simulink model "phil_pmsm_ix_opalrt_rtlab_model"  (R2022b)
settings: Solver=ode3  StartTime=0.0  StopTime=inf  FixedStep=Ts  RelTol=1e-3
PostLoadFcn:
  | phil_pmsm_ix_opalrt_rtlab_param;
InitFcn:
  | phil_pmsm_ix_opalrt_rtlab_param;
undefined symbols (not defined in the file or in its folder): af15, arm1_g1, Boost2lvl_SFun, boost_I, boost_V, C, c62c8459, DB, EFPGASIMConfig, eHSBuildReport, eHSx64_Gen4_Machines_IOConfig1, EX, fault_sw, LABv2024, logs, matlab, Min, models, ns, OPAL, phil_pmsm_ix_opalrt_rtlab, phil_pmsm_ix_opalrt_rtlab_ehs, phil_pmsm_ix_opalrt_rtlab_model, phil_pmsm_ix_opalrt_rtlab_param, RT, Step, TE0741_4, Time, Users, v1, vin, vsrc1, vsrc2, vsrc3
libraries: opal_lib x3, rtlab x2, rtio_opalrt_common x1, ehsSchematicEditorSourceLib x1

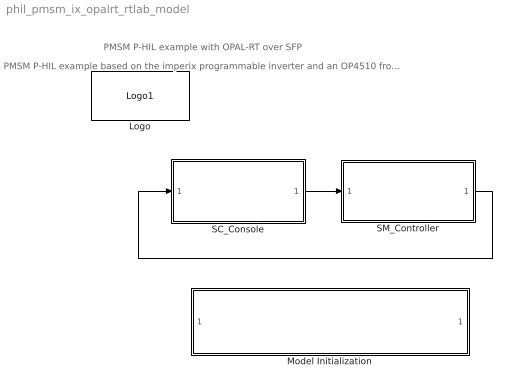
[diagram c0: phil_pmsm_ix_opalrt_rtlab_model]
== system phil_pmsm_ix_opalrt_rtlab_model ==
  note: PMSM P-HIL example based on the imperix programmable inverter and an OP4510 from OPAL-RT.
  note: PMSM P-HIL example with OPAL-RT over SFP
  Logo : opal_lib/Logo1  vide=[]
  Model Initialization : Subsystem  mask(Model Functions){InitFcnX=phil_pmsm_ix_opalrt_rtlab_param;, prel=off, posl=on, inif=on, strf=off}
      mask prompts: InitFcnX "Initialisation"; prel "Preload Function"; posl "PostLoad Function"; inif "InitFcn"; strf "StartFcn"
      mask init:
      | currentBlock = gcb;
      | root = bdroot(currentBlock);
      | 
      | if ~strcmp(get_param(root,'BlockDiagramType'),'library')
      |     if prel==1
      |         set_param(root, 'PreLoadFcn', InitFcnX);
      |     else
      |         set_param(root, 'PreLoadFcn', '');
      |     end
      |     if inif==1
      |         set_param(root, 'InitFcn', InitFcnX);
      |     else
      |         set_param(root, 'InitFcn', '');
      |     end
      |     if strf==1
      |         set_param(root, 'StartFcn', InitFcnX);
      |     else
      |         set_param(root, 'StartFcn', '');
      |     end
      |     if posl==1
      |         set_param(root, 'PostLoadFcn', InitFcnX);
      |     else
      |         set_param(root, 'PostLoadFcn', '');
      |     end
      | end
      | 
      | pos = get_param(currentBlock, 'Position');
      | width = pos(3) - pos(1); height = pos(4) - pos(2);
      | txt = [ upper(root) '\n' '- InitFcn. . . . . '  get_param(root, 'InitFcn') ];
  SC_Console : Subsystem
  SM_Controller : Subsystem
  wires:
  SC_Console/1(to_eHS) -> SM_Controller/1(to_eHS)
  SM_Controller/1(from_eHS) -> SC_Console/1(from_eHS)

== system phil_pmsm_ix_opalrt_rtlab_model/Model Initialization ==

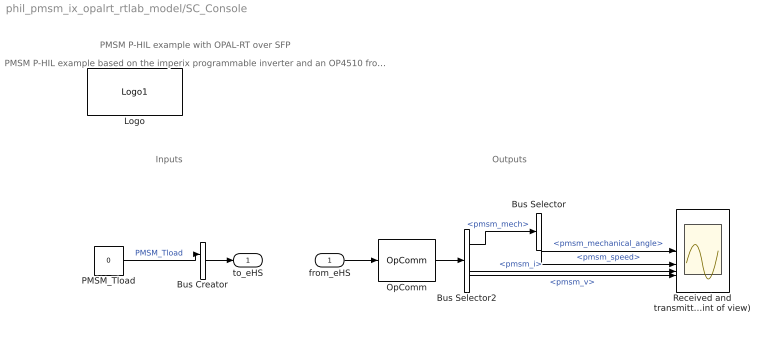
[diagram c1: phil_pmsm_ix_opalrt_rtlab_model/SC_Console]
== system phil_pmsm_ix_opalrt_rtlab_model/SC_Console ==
  note: Inputs
  note: Outputs
  note: PMSM P-HIL example with OPAL-RT over SFP
  note: PMSM P-HIL example based on the imperix programmable inverter and an OP4510 from OPAL-RT.
  from_eHS : Inport  OutDataTypeStr=double
  Bus Creator : BusCreator  Inputs=1
  Bus Selector : BusSelector  OutputSignals=pmsm_mechanical_angle,pmsm_speed
  Bus Selector2 : BusSelector  OutputSignals=pmsm_mech,pmsm_i,pmsm_v
  Logo : opal_lib/Logo1  vide=[]
  OpComm : rtlab/OpComm  nbport=1  groupe_acq=1  subsys_rate=0  st=0  Synchronization=off  Interpolation=off  Threshold=1.0  Missed_Data=off  Sim_Time=off  Samples=off  dynSigOut=off  from_console=0  warning_done=off  writeOpCommFile=off
  PMSM_Tload : Constant  Value=0
  Received and transmitted signals (OP4510 point of view) : Scope  NumInputPorts=4
  to_eHS : Outport  VectorParamsAs1DForOutWhenUnconnected=off
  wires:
  from_eHS/1 -> OpComm/1
  Bus Creator/1 -> to_eHS/1
  OpComm/1 -> Bus Selector2/1
  PMSM_Tload/1 -> Bus Creator/1  "PMSM_Tload"
  Bus Selector2/1 -> Bus Selector/1  "<pmsm_mech>"
  Bus Selector2/2 -> Received and transmitted signals (OP4510 point of view)/3  "<pmsm_i>"
  Bus Selector2/3 -> Received and transmitted signals (OP4510 point of view)/4  "<pmsm_v>"
  Bus Selector/1 -> Received and transmitted signals (OP4510 point of view)/1  "<pmsm_mechanical_angle>"
  Bus Selector/2 -> Received and transmitted signals (OP4510 point of view)/2  "<pmsm_speed>"

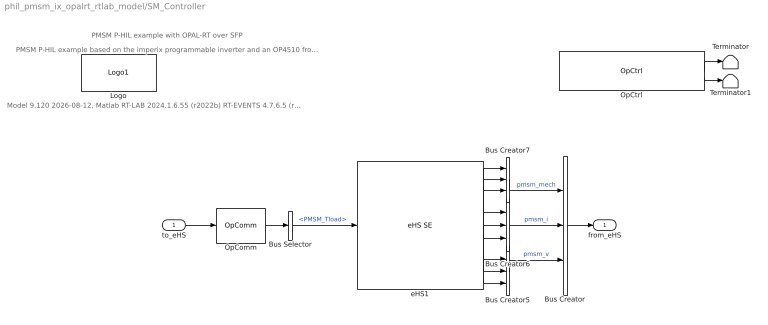
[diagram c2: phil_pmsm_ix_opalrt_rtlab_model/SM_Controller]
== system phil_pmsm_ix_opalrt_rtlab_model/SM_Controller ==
  note: Model 9.120 2026-08-12, Matlab RT-LAB 2024.1.6.55 (r2022b) RT-EVENTS 4.7.6.5 (r2022b.x) eFPGAsim () &copy; 2026 Opal-RT Technologies Inc.
  note: PMSM P-HIL example based on the imperix programmable inverter and an OP4510 from OPAL-RT.
  note: PMSM P-HIL example with OPAL-RT over SFP
  to_eHS : Inport
  Bus Creator{,5..7} (4 alike) : BusCreator  Inputs=3
  Bus Selector : BusSelector  OutputSignals=PMSM_Tload
  Logo : opal_lib/Logo1  vide=[]
  OpComm : rtlab/OpComm  nbport=1  groupe_acq=1  subsys_rate=0  st=0  Synchronization=on  Interpolation=on  Threshold=1.0  Missed_Data=off  Sim_Time=off  Samples=off  dynSigOut=off  from_console=1  warning_done=off  writeOpCommFile=off
  OpCtrl : rtio_opalrt_common/OpCtrl  CtrlName='OpCtrl'  boardid=0  BitstreamFilename=TE0741_4-EX-0001-3_11_2_12-eHSx64_Gen4_Machines_IOConfig1-DB-4A.bin  numconfig=-1  mode=Master  externalClock=off  decimRtsi=0  calibIO=off  SampleTime=0  loadinport=-1  BoardType=TE0741  SecondaryPresent=off  sync_type=Audio  scope_enable=off  fsdFileName=TE0741_4-EX-0001-3_11_2_12-eHSx64_Gen4_Machines_IOConfig1-DB-4A.fsd  mismatch_disable=on
  Terminator : Terminator
  Terminator1 : Terminator
  eHS1 : ehsSchematicEditorSourceLib/eHS SE  modelName=Boost2lvl_SFun - v1  modelUuid=c62c8459-3f79-48c0-af15-759a73c628dc  modelDisplayName=Boost2lvl_SFun  lastLoadedModelText=Circuit loaded on 09-Oct-2024 14:20:43  lastLoadedModelName=Boost2lvl_SFun - v1  lastLoadedModelUuid=c62c8459-3f79-48c0-af15-759a73c628dc  lastLoadedModelDisplayName=Boost2lvl_SFun - v1  triggerUpdate=off  timeStepInfo=Time Step: 230 ns (Min: 230 ns)  inputPins=arm1_g1,fault_sw,vin,vsrc1,vsrc2,vsrc3  outputPins=2Lvl_Ia,2Lvl_Ib,2Lvl_Ic,2Lvl_Va,2Lvl_Vb,2Lvl_Vc,boost_I,boost_V  loadPassed=1  firmwareName=TE0741_4-EX-0001-3_11_2_12-eHSx64_Gen4_Machines_IOConfig1-DB-4A.bin  driverType=SFUN  ehsEffectiveLicense=x128  migrated=on  opCtrlName='OpCtrl'  autoConfigureFirmware=on  ehsFileName=phil_pmsm_ix_opalrt_rtlab_ehs.ehs3  buildReportFile=C:\Users\matlab\OPAL-RT\RT-LABv2024.1_Workspace2\phil_pmsm_ix_opalrt_rtlab\models\phil_pmsm_ix_opalrt_rtlab_model\EFPGASIMConfig\logs\phil_pmsm_ix_opalrt_rtlab_ehs\logs\eHSBuildReport.txt  displayBlockInfos=|
      | x32
      | Time Step: 205 ns (Min: 205 ns)
  from_eHS : Outport  VectorParamsAs1DForOutWhenUnconnected=off
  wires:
  to_eHS/1 -> OpComm/1
  OpComm/1 -> Bus Selector/1
  Bus Creator/1 -> from_eHS/1
  OpCtrl/1 -> Terminator/1
  OpCtrl/2 -> Terminator1/1
  Bus Creator6/1 -> Bus Creator/2  "pmsm_i"
  Bus Creator5/1 -> Bus Creator/3  "pmsm_v"
  Bus Creator7/1 -> Bus Creator/1  "pmsm_mech"
  Bus Selector/1 -> eHS1/1  "<PMSM_Tload>"
  eHS1/3 -> Bus Creator7/3
  eHS1/4 -> Bus Creator6/1
  eHS1/5 -> Bus Creator6/2
  eHS1/6 -> Bus Creator6/3
  eHS1/7 -> Bus Creator5/1
  eHS1/8 -> Bus Creator5/2
  eHS1/9 -> Bus Creator5/3
  eHS1/2 -> Bus Creator7/2
  eHS1/1 -> Bus Creator7/1
